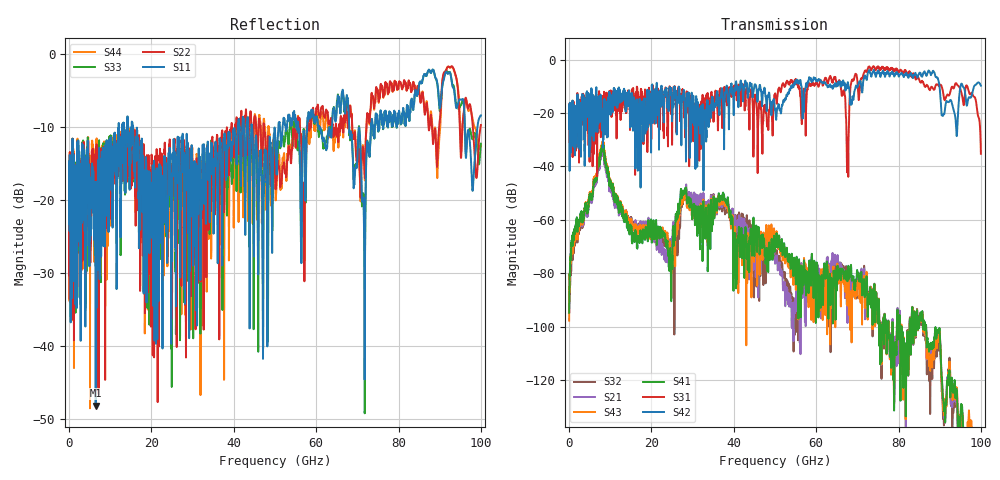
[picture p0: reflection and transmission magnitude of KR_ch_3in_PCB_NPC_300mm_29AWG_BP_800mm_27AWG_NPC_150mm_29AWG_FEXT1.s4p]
# GHz S RI R 45
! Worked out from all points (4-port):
!   4000 points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, 25 MHz to 100 GHz, reference 45 ohm
!   strongest paths, dB at 25 MHz, 25.02 GHz, 50.02 GHz, 75.03 GHz, 100 GHz:
!     S42: -21.2, -20.7, -18.6, -4.1, -9.8
!     S31: -21.2, -31.9, -12.7, -2.5, -35.2
!     S41: -94.8, -75.7, -70.4, -95.7, -140.9
!     S43: -97.8, -75.6, -68.1, -95.6, -139.5
!     S21: -88.9, -66.8, -76.5, -95.5, -145.9
!     S32: -94.8, -69.0, -73.8, -95.5, -144.8
!   lowest |S11| = -48.1 dB at 6.475 GHz (marker M1), VSWR 1.01, Z = 45 - j0.353 ohm
!   |S11| at or under -10 dB: start of sweep to 12.07 GHz; 15.43 GHz to 40.98 GHz (25.55 GHz wide, 90.6 % of centre); 44.42 GHz to 50.82 GHz (6.398 GHz wide, 13.4 % of centre)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
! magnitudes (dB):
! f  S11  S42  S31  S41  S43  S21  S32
! 25 MHz  -16.7  -21.2  -21.2  -94.8  -97.8  -88.9  -94.8
! 6.475 GHz  -48.1  -14.2  -24.1  -45.5  -44.5  -46.7  -45.3
! 24.6 GHz  -18.2  -12.8  -12.2  -72.3  -70.5  -67.6  -67.9
! 63.42 GHz  -11.0  -9.3  -6.1  -83.4  -96.8  -77.5  -85.9
! 67.6 GHz  -6.0  -8.9  -31.9  -83.1  -92.2  -98.6  -85.3
! 76.22 GHz  -10.0  -4.1  -2.7  -103.1  -102.9  -102.2  -102.7
! 100 GHz  -8.4  -9.8  -35.2  -140.9  -139.5  -145.9  -144.8
